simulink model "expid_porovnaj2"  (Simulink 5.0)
settings: Solver=ode5  StartTime=0.0  StopTime=500  FixedStep=0.1  RelTol=1e-3

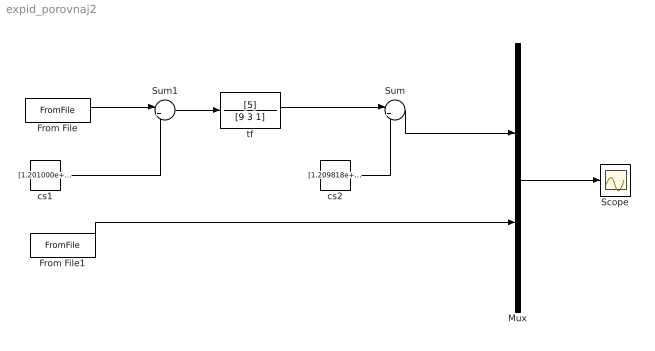
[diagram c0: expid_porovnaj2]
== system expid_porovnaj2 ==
  From File : FromFile  FileName=vstup_u.mat  SampleTime=0
  From File1 : FromFile  FileName=vstup_y.mat  SampleTime=0
  Mux : Mux  Inputs=2
  Scope : Scope
  Sum : Sum  Inputs=|++
  Sum1 : Sum  Inputs=|+-
  cs1 : Constant  Value=[1.201000e+001]
  cs2 : Constant  Value=[1.209818e+002]
  tf : TransferFcn  Numerator=[5]  Denominator=[9 3 1]
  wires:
  cs2/1 -> Sum/2
  Sum/1 -> Mux/1
  From File1/1 -> Mux/2
  From File/1 -> Sum1/1
  Sum1/1 -> tf/1
  cs1/1 -> Sum1/2
  Mux/1 -> Scope/1
  tf/1 -> Sum/1
